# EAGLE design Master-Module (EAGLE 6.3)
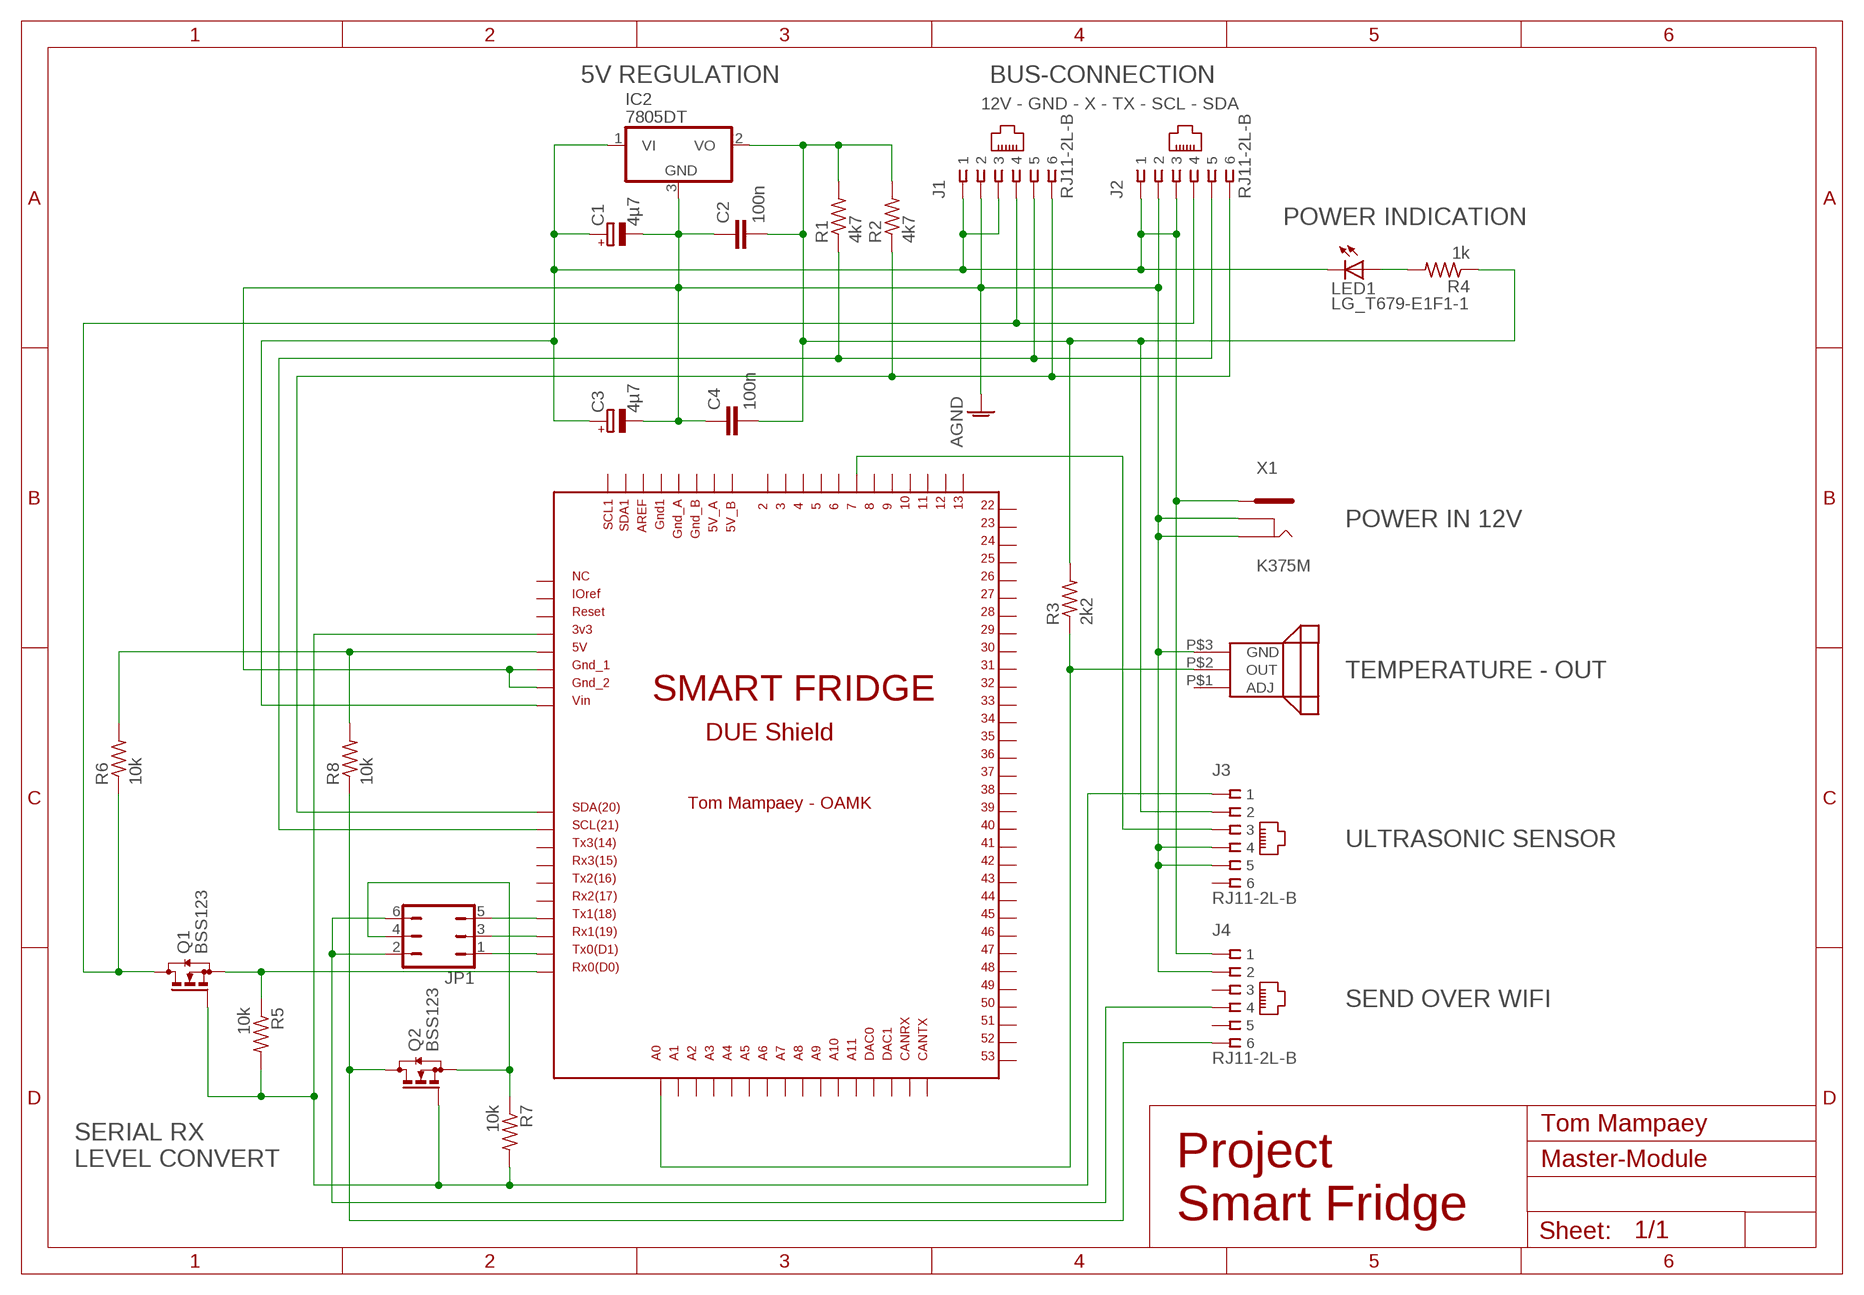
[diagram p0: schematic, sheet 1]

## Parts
C1  4µ7  CPOL-EUB  [PANASONIC_B]
C2  100n  C-EUC0603  [C0603]
C3  4µ7  CPOL-EUB  [PANASONIC_B]
C4  100n  C-EUC0603  [C0603]
IC2  7805DT  [TO252]
J1  RJ11-2L-B  [RJ11-NO_SHIELD]
J2  RJ11-2L-B  [RJ11-NO_SHIELD]
J3  RJ11-2L-B  [RJ11-NO_SHIELD]
J4  RJ11-2L-B  [RJ11-NO_SHIELD]
JP1  JP3Q  [JP3Q]
LED1  LG_T679-E1F1-1  [PLCC2]
Q1  BSS123  [SOT23]
Q2  BSS123  [SOT23]
R1  4k7  R-US_R0402  [R0402]
R2  4k7  R-US_R0402  [R0402]
R3  2k2  R-US_R0402  [R0402]
R4  1k  R-US_R0402  [R0402]
R5  10k  R-US_R0402  [R0402]
R6  10k  R-US_R0402  [R0402]
R7  10k  R-US_R0402  [R0402]
R8  10k  R-US_R0402  [R0402]
U$1  DUE(NORMAL)  [DUE(NORMAL)]
U$2  LM335  [LM335]
X1  K375M  [K375M]

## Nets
AGND: C1.- C2.1 C3.- C4.1 IC2.3(GND) J1.2 J2.2 J3.4 J3.5 J4.2 U$1.GND_1 U$1.GND_2 U$2.P$3(GND) X1.P$1 X1.P$6
N$1: J1.6 J2.6 R2.1 U$1.SDA
N$2: J1.4 J2.4 Q1.3(D) R6.1
N$3: J1.5 J2.5 R1.1 U$1.SCL
N$4: R6.2 R8.2 U$1.5V
N$5: R3.1 U$1.A0 U$2.P$2(OUT)
N$6: J3.3 U$1.7
N$7: LED1.A R4.2
N$8: C2.2 C4.2 IC2.2(VO) J3.2 R1.2 R2.2 R3.2 R4.1
N$9: Q1.2(S) R5.1 U$1.RX0
N$10: C1.+ C3.+ IC2.1(VI) J1.1 J1.3 J2.1 J2.3 J4.1 LED1.C U$1.VIN X1.P$7
N$11: JP1.1 U$1.TX0
N$14: J3.1 Q1.1(G) Q2.1(G) R5.2 R7.2 U$1.3V3
N$30: JP1.3 U$1.RX1
N$31: JP1.5 U$1.TX1
N$33: J4.4 JP1.2 JP1.6
N$34: J4.6 Q2.3(D) R8.1
N$35: JP1.4 Q2.2(S) R7.1
Unconnected: J3.6 J4.3 J4.5 U$1.2 U$1.3 U$1.4 U$1.5 U$1.5V_A U$1.5V_B U$1.6 U$1.8 U$1.9 U$1.10 U$1.11 U$1.12 U$1.13 U$1.22 U$1.23 U$1.24 U$1.25 U$1.26 U$1.27 U$1.28 U$1.29 U$1.30 U$1.31 U$1.32 U$1.33 U$1.34 U$1.35 U$1.36 U$1.37 U$1.38 U$1.39 U$1.40 U$1.41 U$1.42 U$1.43 U$1.44 U$1.45 U$1.46 U$1.47 U$1.48 U$1.49 U$1.50 U$1.51 U$1.52 U$1.53 U$1.A1 U$1.A2 U$1.A3 U$1.A4 U$1.A5 U$1.A6 U$1.A7 U$1.A8 U$1.A9 U$1.A10 U$1.A11 U$1.AREF U$1.CANRX U$1.CANTX U$1.DAC0 U$1.DAC1 U$1.GND1 U$1.GND_A U$1.GND_B U$1.IOREF U$1.NC U$1.RESET U$1.RX2 U$1.RX3 U$1.SCL1 U$1.SDA1 U$1.TX2 U$1.TX3 U$2.P$1(ADJ)

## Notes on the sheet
- 5V REGULATION | BUS-CONNECTION
- 12V - GND - X - TX - SCL - SDA
- POWER INDICATION
- POWER IN 12V
- TEMPERATURE - OUT
- ULTRASONIC SENSOR
- SEND OVER WIFI
- Tom Mampaey
- SERIAL RX 
  LEVEL CONVERT
- Project 
  Smart Fridge

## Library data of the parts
C1 C3 = resistor:CPOL-EU: POLARIZED CAPACITOR, European symbol
C2 C4 = resistor:C-EU: CAPACITOR, European symbol
IC2 = linear:78*: Positive VOLTAGE REGULATOR Source: http://cache.national.com/ds/LM/LM78L05.pdf http://www.fairchildsemi.com/ds/LM/LM7805.pdf
J1-J4 = con-tycoelectronics:RJ11: CORCOM Modular RJ Jacks No Shield Source: www.tycoelectronics.com .. ENG_DS_1654001_1099_RJ_L_0507.pdf; MF: TYCO ELECTRONICS; MPN: RJ11-2L-B; OC_FARNELL: unknown; OC_NEWARK: 83F4463
JP1 = jumper:JP3Q: JUMPER
LED1 = led:*_T679-?-1: LC TOPLED® Low Current LED; COLOR: green
Q1 Q2 = transistor-small-signal:BSS123: N-CHANNEL MOS FET
R1-R8 = rcl:R-US_: RESISTOR, American symbol
U$1 = DUE-shield custom:DUE(NORMAL)
U$2 = LM335:LM335
X1 = con-power c:K375M: K375M - DC POWER JACK 2.5mm/CENTRAL PIN Source: Data sheet

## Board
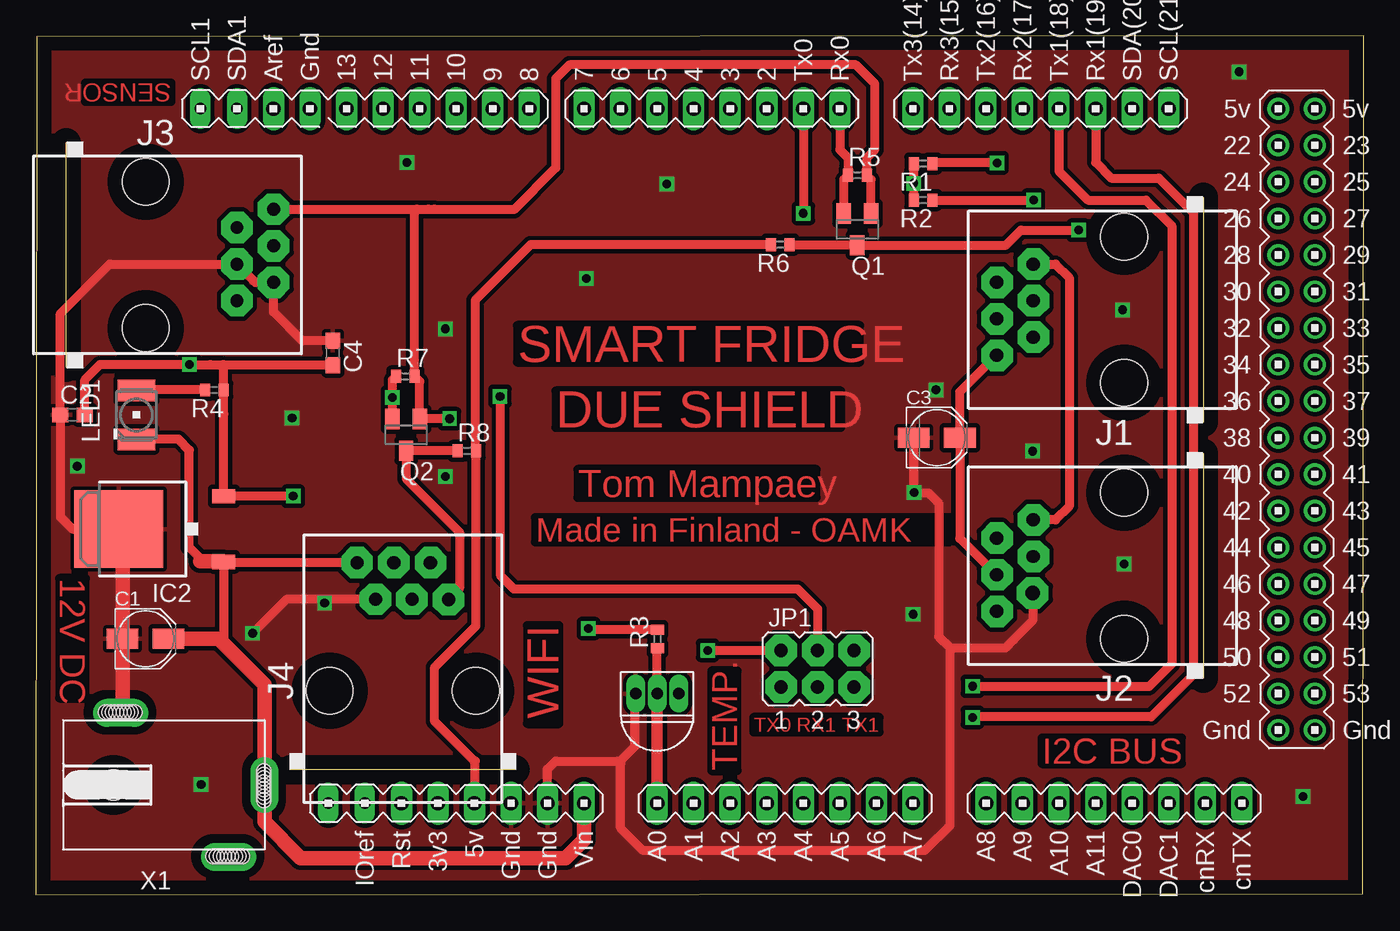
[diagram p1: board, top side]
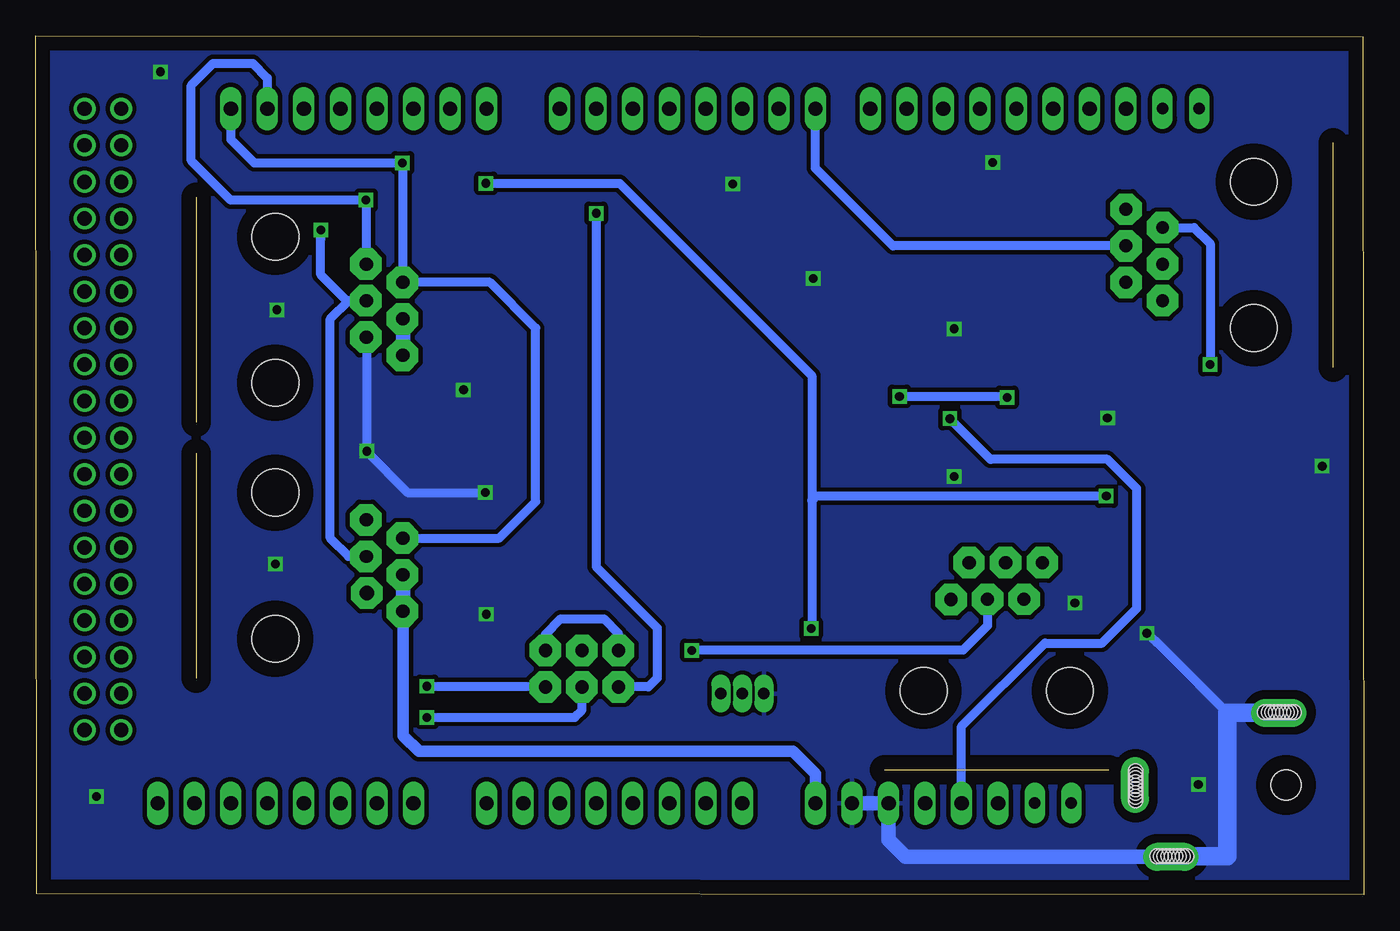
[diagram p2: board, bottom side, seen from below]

Size 92.28 x 59.66 mm. Coordinates in mm from the lower left corner, seen from the top.
Outline: 0,0 92.23,0.05 92.28,59.66 0.05,59.61 0,0
Copper layers (1*16): Top 0.035mm / dielectric 1.5mm / Bottom 0.035mm
Design rules "default": minimum track width 10mil, minimum drill 24mil, track to track 8mil, track to pad 8mil, pad to pad 8mil, via to via 8mil, smd to smd 8mil, copper to edge 40mil, drill to drill 8mil, minimum pad ring 10mil, minimum via ring 8mil, stop-mask expansion 4mil, vias tented up to drill 0mil, thermal gap 10mil

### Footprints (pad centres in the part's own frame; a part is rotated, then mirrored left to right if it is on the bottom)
PANASONIC_B = smd 2.2 x 1.4: + 1.6,0; - -1.6,0
C0603 = smd 1.1 x 1: 1 -0.85,0; 2 0.85,0
TO252 = smd 1 x 1.6: 1 -2.28,-4.8; 2 2.28,-4.8 | smd 5.4 x 6.2: 3 0,2.5
RJ11-NO_SHIELD = drill 0.9 pad 1.4: 1 -3.175,8.89; 2 -1.905,6.35; 3 -0.635,8.89; 4 0.635,6.35; 5 1.905,8.89; 6 3.175,6.35 | hole 3.251: -5.08,0; 5.08,0
JP3Q = drill 0.914 octagon: 1 -2.54,-1.27; 2 -2.54,1.27; 3 0,-1.27; 4 0,1.27; 5 2.54,-1.27; 6 2.54,1.27
PLCC2 = smd 2.6 x 1.5: A 0,1.7; C 0,-1.7
SOT23 = smd 1 x 1.4: 1 -0.95,-1.1; 2 0.95,-1.1; 3 0,1.1
R0402 = smd 0.7 x 0.9: 1 -0.65,0; 2 0.65,0
DUE(NORMAL) = drill 1 long: 2 -1.27,22.86; 3 -3.81,22.86; 3V3 -24.13,-25.4; 4 -6.35,22.86; 5 -8.89,22.86; 5V -21.59,-25.4; 6 -11.43,22.86; 7 -13.97,22.86; 8 -17.78,22.86; 9 -20.32,22.86; 10 -22.86,22.86; 11 -25.4,22.86; 12 -27.94,22.86; 13 -30.48,22.86; A0 -8.89,-25.4; A1 -6.35,-25.4; A2 -3.81,-25.4; A3 -1.27,-25.4; A4 1.27,-25.4; A5 3.81,-25.4; A6 6.35,-25.4; A7 8.89,-25.4; A8 13.97,-25.4; A9 16.51,-25.4; A10 19.05,-25.4; A11 21.59,-25.4; AREF -35.56,22.86; AREF1 -35.56,22.86; CANRX 29.21,-25.4; CANTX 31.75,-25.4; DAC0 24.13,-25.4; DAC1 26.67,-25.4; GND1 -33.02,22.86; GND_1 -19.05,-25.4; GND_2 -16.51,-25.4; RESET -26.67,-25.4; RX0 3.81,22.86; RX1 21.59,22.86; RX2 16.51,22.86; RX3 11.43,22.86; SCL 26.67,22.86; SDA 24.13,22.86; TX0 1.27,22.86; TX1 19.05,22.86; TX2 13.97,22.86; TX3 8.89,22.86; VIN -13.97,-25.4 | drill 1: 5V_A 34.29,22.86; 5V_B 36.83,22.86; 22 34.29,20.32; 23 36.83,20.32; 24 34.29,17.78; 25 36.83,17.78; 26 34.29,15.24; 27 36.83,15.24; 28 34.29,12.7; 29 36.83,12.7; 30 34.29,10.16; 31 36.83,10.16; 32 34.29,7.62; 33 36.83,7.62; 34 34.29,5.08; 35 36.83,5.08; 36 34.29,2.54; 37 36.83,2.54; 38 34.29,0; 39 36.83,0; 40 34.29,-2.54; 41 36.83,-2.54; 42 34.29,-5.08; 43 36.83,-5.08; 44 34.29,-7.62; 45 36.83,-7.62; 46 34.29,-10.16; 47 36.83,-10.16; 48 34.29,-12.7; 49 36.83,-12.7; 50 34.29,-15.24; 51 36.83,-15.24; 52 34.29,-17.78; 53 36.83,-17.78; GND_A 34.29,-20.32; GND_B 36.83,-20.32 | drill 0.8 pad 1.422 long: IOREF -29.21,-25.4; NC -31.75,-25.4; SCL1 -40.64,22.86; SDA1 -38.1,22.86
LM335 = drill 0.8 long: P$1 0,1.5; P$2 0,0; P$3 0,-1.5
K375M = drill 1 pad 1.93 long: P$1 5,3; P$6 -5,-4.5; P$7 0.004,-7.007 | hole 2.1: 0,3.5 | hole 1: -4.953,-3.429; -4.953,-3.683; -4.953,-3.937; -4.953,-4.191; -4.953,-4.445; -4.953,-4.699; -4.953,-4.953; -4.953,-5.207; -4.953,-5.461; -1.067,-6.96; -0.813,-6.96; -0.559,-6.96; -0.305,-6.96; -0.051,-6.96; 0.203,-6.96; 0.457,-6.96; 0.711,-6.96; 0.965,-6.96; 5.055,4.064; 5.055,3.81; 5.055,3.556; 5.055,3.302; 5.055,3.048; 5.055,2.794; 5.055,2.54; 5.055,2.286; 5.055,2.032

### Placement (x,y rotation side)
C1  7.62,17.78 0 top
C2  2.54,33.34 0 top
C3  62.62,31.75 0 top
C4  20.64,37.63 270 top
IC2  8.26,25.4 90 top
J1  75.64,40.64 90 top
J2  75.64,22.86 90 top
J3  7.62,44.45 270 top
J4  25.5,14.17 0 top
JP1  54.33,15.7 0 top
LED1  6.99,33.34 0 top
Q1  57.1,46.23 180 top
Q2  25.73,31.95 180 top
R1  61.67,50.8 180 top
R2  61.67,48.26 180 top
R3  43.21,17.75 90 top
R4  12.41,35.06 180 top
R5  57.1,49.99 0 top
R6  51.74,45.16 180 top
R7  25.68,36.02 0 top
R8  29.95,30.84 0 top
U$1  52.07,31.75 0 top
U$2  43.18,13.97 270 top
X1  8.89,7.62 90 top

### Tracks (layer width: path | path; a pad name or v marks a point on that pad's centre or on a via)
AGND  (via drill 0.6)
  Top 0.61: C3.- 61.04,31.74 v61.04,27.94 61.01,27.91 62.03,27.91 62.76,27.18 62.76,17.93 63.55,17.14 | IC2.3 2.54,25.4 1.69,26.25 C2.1 1.69,40.37 5.13,43.81 J3.4 15.24,42.55 J3.5 16.51,40.49 18.52,38.48 C4.1 | 40.64,9.09 40.64,4.62 42.22,3.05 61.77,3.05 63.55,4.83 63.55,17.14 | 40.64,9.09 40.64,9.3 41.66,10.31 41.66,13.95 U$2.P$3 | 63.55,17.14 67.39,17.14 67.41,17.17 67.94,17.7 69.29,19.05 J2.2 | U$1.GND_2 35.56,8.71 36.12,9.27 40.46,9.27 40.64,9.09 | J4.2 17.42,20.52 v15.06,18.16
  Top 1.016: X1.P$1 6.02,12.75 C1.- 6.02,24.43 6.99,25.4 IC2.3
  Bottom 0.61: J1.2 69.29,30.8 66.43,27.94 v61.04,27.94 | v15.06,18.16 14.38,17.53 9.47,12.62
  Bottom 1.016: U$1.GND_2 U$1.GND_1 33.02,3.81 31.83,2.62 X1.P$6 13.31,2.54
  Bottom 1.27: X1.P$1 9.47,12.62 9.47,2.67 13.39,2.67 X1.P$6
  other vias: 69.29,30.81 25.78,50.88 43.84,49.38 28.45,39.32 17.81,33.12 88.09,6.81 60.99,19.48 75.64,22.96 75.54,40.64 11.48,7.65 83.64,57.18 38.25,42.82 20.07,20.27 2.87,29.77 62.56,35.08 28.45,29.06
  pour Bottom (isolate 0.305): 92.23,59.59 92.23,0.05 0.05,0.05 0.05,59.59 0.1,59.59
  pour Top (isolate 0.305): 0.05,59.61 92.23,59.61 92.23,0.05 0.05,0.05
N$1  (via drill 0.6)
  Top 0.61: R2.1 v69.34,48.26 | J1.6 70.88,43.81 71.83,42.86 71.83,26.99 70.88,26.04 J2.6
  Bottom 0.61: U$1.SDA 76.2,56.74 77.22,57.76 79.96,57.76 81.48,56.24 81.48,51 78.74,48.26 v69.34,48.26 69.29,48.21 J1.6
N$2  (via drill 0.6)
  Top 0.61: v72.47,46.18 68.48,46.18 67.43,45.13 Q1.3 52.56,45.13 R6.1
  Bottom 0.61: J2.4 70.56,23.5 71.83,24.77 71.83,40.01 70.56,41.27 | J1.4 70.56,41.27 | 70.56,41.27 70.69,41.27 72.49,43.08 72.49,45.54 v72.47,46.18
N$3  (via drill 0.6)
  Top 0.61: v66.8,50.85 62.37,50.85 R1.1
  Bottom 0.61: J2.5 60.08,24.77 57.54,27.3 57.54,39.37 60.72,42.55 J1.5 66.75,50.8 v66.8,50.85 77.11,50.85 78.74,52.48 U$1.SCL
N$4
  Top 0.61: U$1.5V 30.53,6.4 30.53,9.3 30.45,9.3 27.71,12.04 27.71,15.8 30.58,18.67 30.58,30.82 R8.2 30.53,30.9 30.53,41.3 34.39,45.16 R6.2
N$5
  Top 0.61: U$2.P$2 43.18,17.08 R3.1
  Top 0.813: U$1.A0 U$2.P$2
N$6
  Bottom 0.61: J3.3 32.7,45.09 38.1,50.48 U$1.7
N$7
  Top 0.61: R4.2 7.01,35.06 LED1.A
N$8  (via drill 0.6)
  Top 0.61: C2.2 3.39,35.77 4.45,36.83 v10.67,36.83 13.03,36.83 | 13.03,36.83 13.02,35.88 13.02,34.94 R4.1 13.05,33.39 IC2.2 v17.88,27.69 | 12.12,36.83 13.03,36.83 | R1.2 R2.2 61.02,49.42 60.96,49.48 61.01,49.58 v61.01,49.43 | 38.48,18.41 v38.41,18.49 38.49,18.41 R3.2 | C4.2 13.08,36.78 13.03,36.83
  Bottom 0.61: v61.01,49.43 51.71,49.43 38.35,36.07 38.35,27.38 | 38.35,27.38 38.35,18.54 v38.41,18.49 | v17.88,27.69 38.05,27.69 38.35,27.38 | J3.2 11.79,46.35 10.67,45.24 v10.67,36.83
N$9
  Top 0.61: Q1.2 56.15,49.69 R5.1 56.44,51.21 55.88,51.77 U$1.RX0
N$10
  Top 0.61: J2.3 64.22,24.75 C3.+ 64.22,34.94 J1.1 | 12.95,17.53 13.05,17.63 IC2.1 13.05,23.06 J4.1 | 11.43,23.18 11.43,23.37 10.67,24.13 10.67,30.89 9.91,31.65 LED1.C
  Top 1.016: U$1.VIN 38.1,3.81 36.83,2.54 18.41,2.54 15.9,5.06 X1.P$7 15.9,14.58 12.95,17.53 12.7,17.78 C1.+ | 11.43,23.18 13,23.18 IC2.1
  Bottom 0.813: U$1.VIN 38.1,8.38 39.67,9.96 65.66,9.96 66.75,11.05 J2.1
  Bottom 1.016: J1.1 J1.3 | J2.1 J2.3
N$11  (via drill 0.6)
  Top 0.61: U$1.TX0 v53.34,47.35
  Bottom 0.61: v53.34,47.35 53.34,22.78 49.1,18.54 49.1,15.04 49.71,14.43 JP1.1
N$12  (via drill 0.9 pad 2.18)
  other vias: 13.97,46.35
N$13  (via drill 0.9 pad 2.18)
  other vias: 16.51,45.09
N$14  (via drill 0.6, 0.9 pad 2.18)
  Top 0.61: J3.1 26.47,47.62 | 26.47,47.62 27.28,47.62 | 27.28,47.62 27.69,47.62 | Q1.1 58.05,49.69 R5.2 57.75,51.2 58.32,51.77 58.32,56.34 57,57.66 37.08,57.66 36.12,56.69 36.12,50.49 33.22,47.6 27.3,47.6 27.28,47.62 | 26.47,47.62 26.33,47.49 R7.2 26.68,35.67 Q2.1 26.7,33.07 v28.75,33.07
  Bottom 0.61: U$1.3V3 27.94,11.68 22.15,17.48 18.19,17.48 15.77,19.89 15.77,28.22 17.8,30.25 25.93,30.25 v28.75,33.07
  other vias: 16.51,47.62
N$15  (via drill 0.9 pad 2.18)
  other vias: 13.97,43.81
N$16  (via drill 0.9 pad 2.18)
  other vias: 16.51,42.55
N$17  (via drill 0.9 pad 2.18)
  other vias: 13.97,41.27
N$18  (via drill 0.9 pad 2.18)
  other vias: 69.34,43.81
N$19  (via drill 0.9 pad 2.18)
  other vias: 66.8,42.55
N$20  (via drill 0.9 pad 2.18)
  other vias: 69.34,41.27
N$21  (via drill 0.9 pad 2.18)
  other vias: 66.8,40.01
N$22  (via drill 0.9 pad 2.18)
  other vias: 66.8,37.47
N$23  (via drill 0.9 pad 2.18)
  other vias: 69.34,26.04
N$24  (via drill 0.9 pad 2.18)
  other vias: 69.34,23.5
N$25  (via drill 0.9 pad 2.18)
  other vias: 66.8,22.23
N$26  (via drill 0.9 pad 2.18)
  other vias: 66.8,19.68
N$27  (via drill 0.9 pad 2.18)
  other vias: 69.34,38.73
N$28  (via drill 0.9 pad 2.18)
  other vias: 66.8,24.77
N$29  (via drill 1 pad 2.18)
  other vias: 69.29,20.95
N$30  (via drill 0.6)
  Top 0.61: U$1.RX1 73.66,50.88 74.75,49.78 78.05,49.78 80.47,47.37 80.47,15.29 77.52,12.34 65.13,12.34 v65.1,12.32
  Bottom 0.61: v65.1,12.32 54.84,12.32 54.33,12.83 JP1.3
N$31  (via drill 0.6)
  Top 0.61: U$1.TX1 71.12,50.27 73.13,48.26 77.17,48.26 78.94,46.48 78.94,16.03 77.37,14.45 65.13,14.45 v65.1,14.48
  Bottom 0.61: v65.1,14.48 56.92,14.48 JP1.5
N$32  (via drill 0.9 pad 2.18)
  other vias: 22.33,23.06
N$33  (via drill 0.6)
  Top 0.61: v46.69,16.97 JP1.2
  Bottom 0.61: JP1.6 56.87,18.09 55.8,19.15 52.81,19.15 51.79,18.14 JP1.2 | J4.4 26.14,18.69 27.84,16.99 46.66,16.99 v46.69,16.97
N$34
  Top 0.61: J4.6 29.44,21.29 29.44,25.2 25.73,28.91 Q2.3 25.75,30.84 R8.1
N$35  (via drill 0.6)
  Top 0.61: Q2.2 v24.78,34.54 24.78,35.77 R7.1 | JP1.4 54.36,16.97 54.36,19.84 52.96,21.23 33.22,21.23 32.31,22.15 32.31,34.42 32.28,34.44 32.28,34.59 v32.26,34.62
  Bottom 0.61: v32.26,34.62 24.86,34.62 v24.78,34.54
N$36  (via drill 0.9 pad 2.18)
  other vias: 24.89,23.06
N$37  (via drill 0.9 pad 2.18)
  other vias: 27.43,23.06
N$38  (via drill 0.9 pad 2.18)
  other vias: 28.68,20.5
N$39  (via drill 0.9 pad 2.18)
  other vias: 26.14,20.52
N$40  (via drill 0.9 pad 2.18)
  other vias: 23.6,20.52
N$41  (via drill 0.9 pad 2.18)
  other vias: 51.79,14.43
N$42  (via drill 0.9 pad 2.18)
  other vias: 51.79,16.97
N$43  (via drill 0.9 pad 2.18)
  other vias: 54.33,16.97
N$44  (via drill 0.9 pad 2.18)
  other vias: 54.33,14.43
N$45  (via drill 0.9 pad 2.18)
  other vias: 56.87,16.97
N$46  (via drill 0.9 pad 2.18)
  other vias: 56.87,14.43

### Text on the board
Top: SENSOR | SMART FRIDGE | DUE SHIELD | Tom Mampaey | Made in Finland - OAMK | 12V DC | WIFI | TX0 RX1 TX1 | TEMP. | I2C BUS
